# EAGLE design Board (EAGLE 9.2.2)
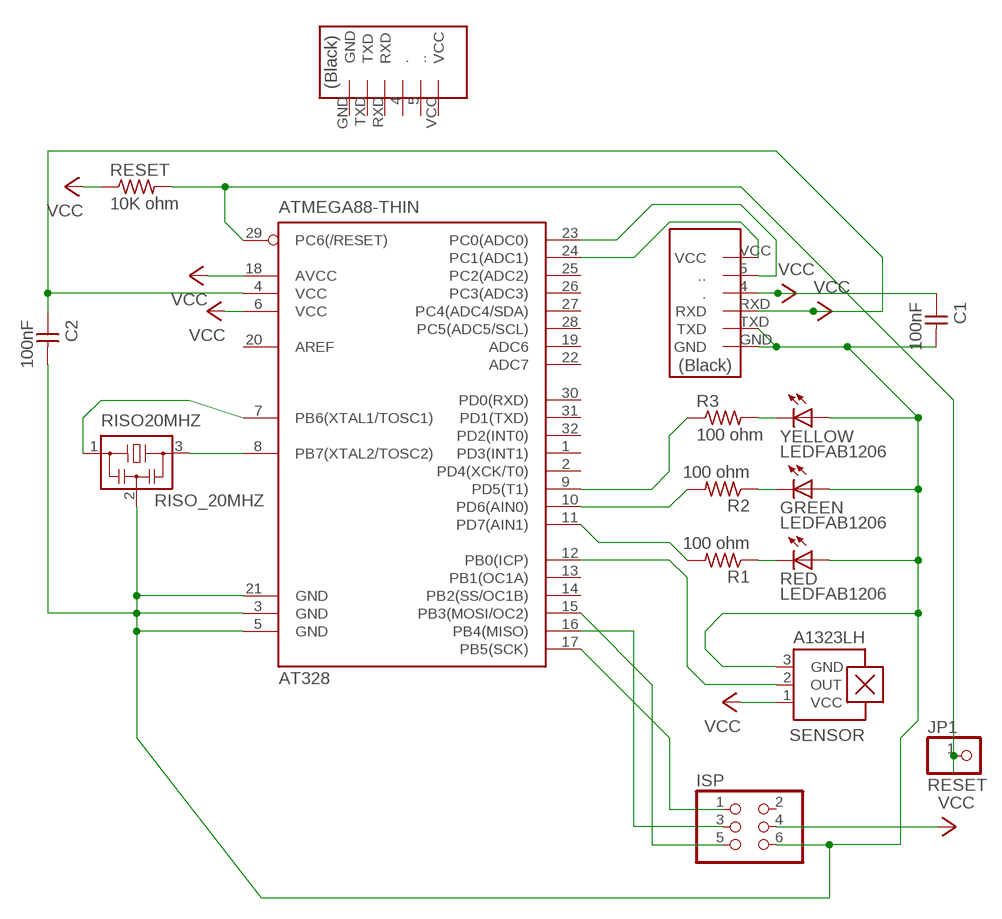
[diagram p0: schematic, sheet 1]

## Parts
AT328  ATMEGA88-THIN  [TQFP32-08THIN]
C1  100nF  CAP-UNPOLARIZEDFAB  [C1206FAB]
C2  100nF  CAP-UNPOLARIZEDFAB  [C1206FAB]
FTDI  FTDI-SMD-HEADER  [1X06SMD]
GREEN  LEDFAB1206  [LED1206FAB]
ISP  PINHD-2X3-SMD  [2X03SMD]
JP1  RESET  PINHD-1X1  [1X01]
R1  100 ohm  RES-US1206FAB  [R1206FAB]
R2  100 ohm  RES-US1206FAB  [R1206FAB]
R3  100 ohm  RES-US1206FAB  [R1206FAB]
RED  LEDFAB1206  [LED1206FAB]
RESET  10K ohm  RES-US1206FAB  [R1206FAB]
RISO20MHZ  RISO_20MHZ  RESONATOR  [EFOBM]
SENSOR  A1323LH  [SOT23-W]
U$1  PINO_FTDI-SMD  [1X06SMD]
YELLOW  LEDFAB1206  [LED1206FAB]

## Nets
GND: AT328.3(GND) AT328.5(GND) AT328.21(GND) C1.2 C2.2 FTDI.GND FTDI.TXD GREEN.1(A) ISP.6(6_GND) RED.1(A) RISO20MHZ.2 SENSOR.3(GND) YELLOW.1(A)
MISO: AT328.16(PB4(MISO)) ISP.3(3_MISO)
MOSI: AT328.15(PB3(MOSI/OC2)) ISP.5(5_MOSI)
N$1: R3.2 YELLOW.2(C)
N$2: R1.1 RED.2(C)
N$3: GREEN.2(C) R2.1
N$4: AT328.11(PD7(AIN1)) R1.2
N$5: AT328.10(PD6(AIN0)) R2.2
N$6: AT328.9(PD5(T1)) R3.1
OUT1: AT328.24(PC1(ADC1)) FTDI.VCC
OUT2: AT328.23(PC0(ADC0)) FTDI.5(..)
OUT_SENSOR: AT328.12(PB0(ICP)) SENSOR.2(OUT)
RESET: AT328.29(PC6(/RESET)) JP1.1 RESET.2
SCK: AT328.17(PB5(SCK)) ISP.1(1_SCK)
VCC: AT328.4(VCC) AT328.6(VCC) AT328.18(AVCC) C1.1 C2.1 FTDI.4(.) FTDI.RXD ISP.4(4_VCC) RESET.1 SENSOR.1(VCC)
XSTAL1: AT328.7(PB6(XTAL1/TOSC1)) RISO20MHZ.1
XSTAL2: AT328.8(PB7(XTAL2/TOSC2)) RISO20MHZ.3
Unconnected: AT328.1(PD3(INT1)) AT328.2(PD4(XCK/T0)) AT328.13(PB1(OC1A)) AT328.14(PB2(SS/OC1B)) AT328.19(ADC6) AT328.20(AREF) AT328.22(ADC7) AT328.25(PC2(ADC2)) AT328.26(PC3(ADC3)) AT328.27(PC4(ADC4/SDA)) AT328.28(PC5(ADC5/SCL)) AT328.30(PD0(RXD)) AT328.31(PD1(TXD)) AT328.32(PD2(INT0)) ISP.2(2_RESET) U$1.4(.) U$1.5(..) U$1.GND U$1.RXD U$1.TXD U$1.VCC

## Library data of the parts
AT328 = fab:ATMEGA88-THIN
C1 C2 = fab:CAP-UNPOLARIZED
FTDI = fab:FTDI-SMD-HEADER
GREEN RED YELLOW = fab:LED: LED
ISP = fab:PINHD-2X3-SMD: PIN HEADER
JP1 = pinhead:PINHD-1X1: PIN HEADER
R1-R3 RESET = fab:RES-US: Resistor (US Symbol)
RISO20MHZ = fab:RESONATOR
SENSOR = allegro:A13*?: Linear Hall Effect Sensor ICs Continuous-Time Ratiometric High-Temperature Operation Programmable Linear with Analog Output A1302 -Replacement- UGN3503 Source: http://www.allegromicro.com/en/Products/Part_Numbers/1301/1301.pdf http://www.allegromicro.com/en/Products/Part_Numbers/1321/1321.pdf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; MF: ALLEGRO MICROSYSTEMS, INC.; MPN: A1323LLHLT-T; OC_FARNELL: 1651968; OC_NEWARK: 65K5152
U$1 = fab:PINO_FTDI-SMD

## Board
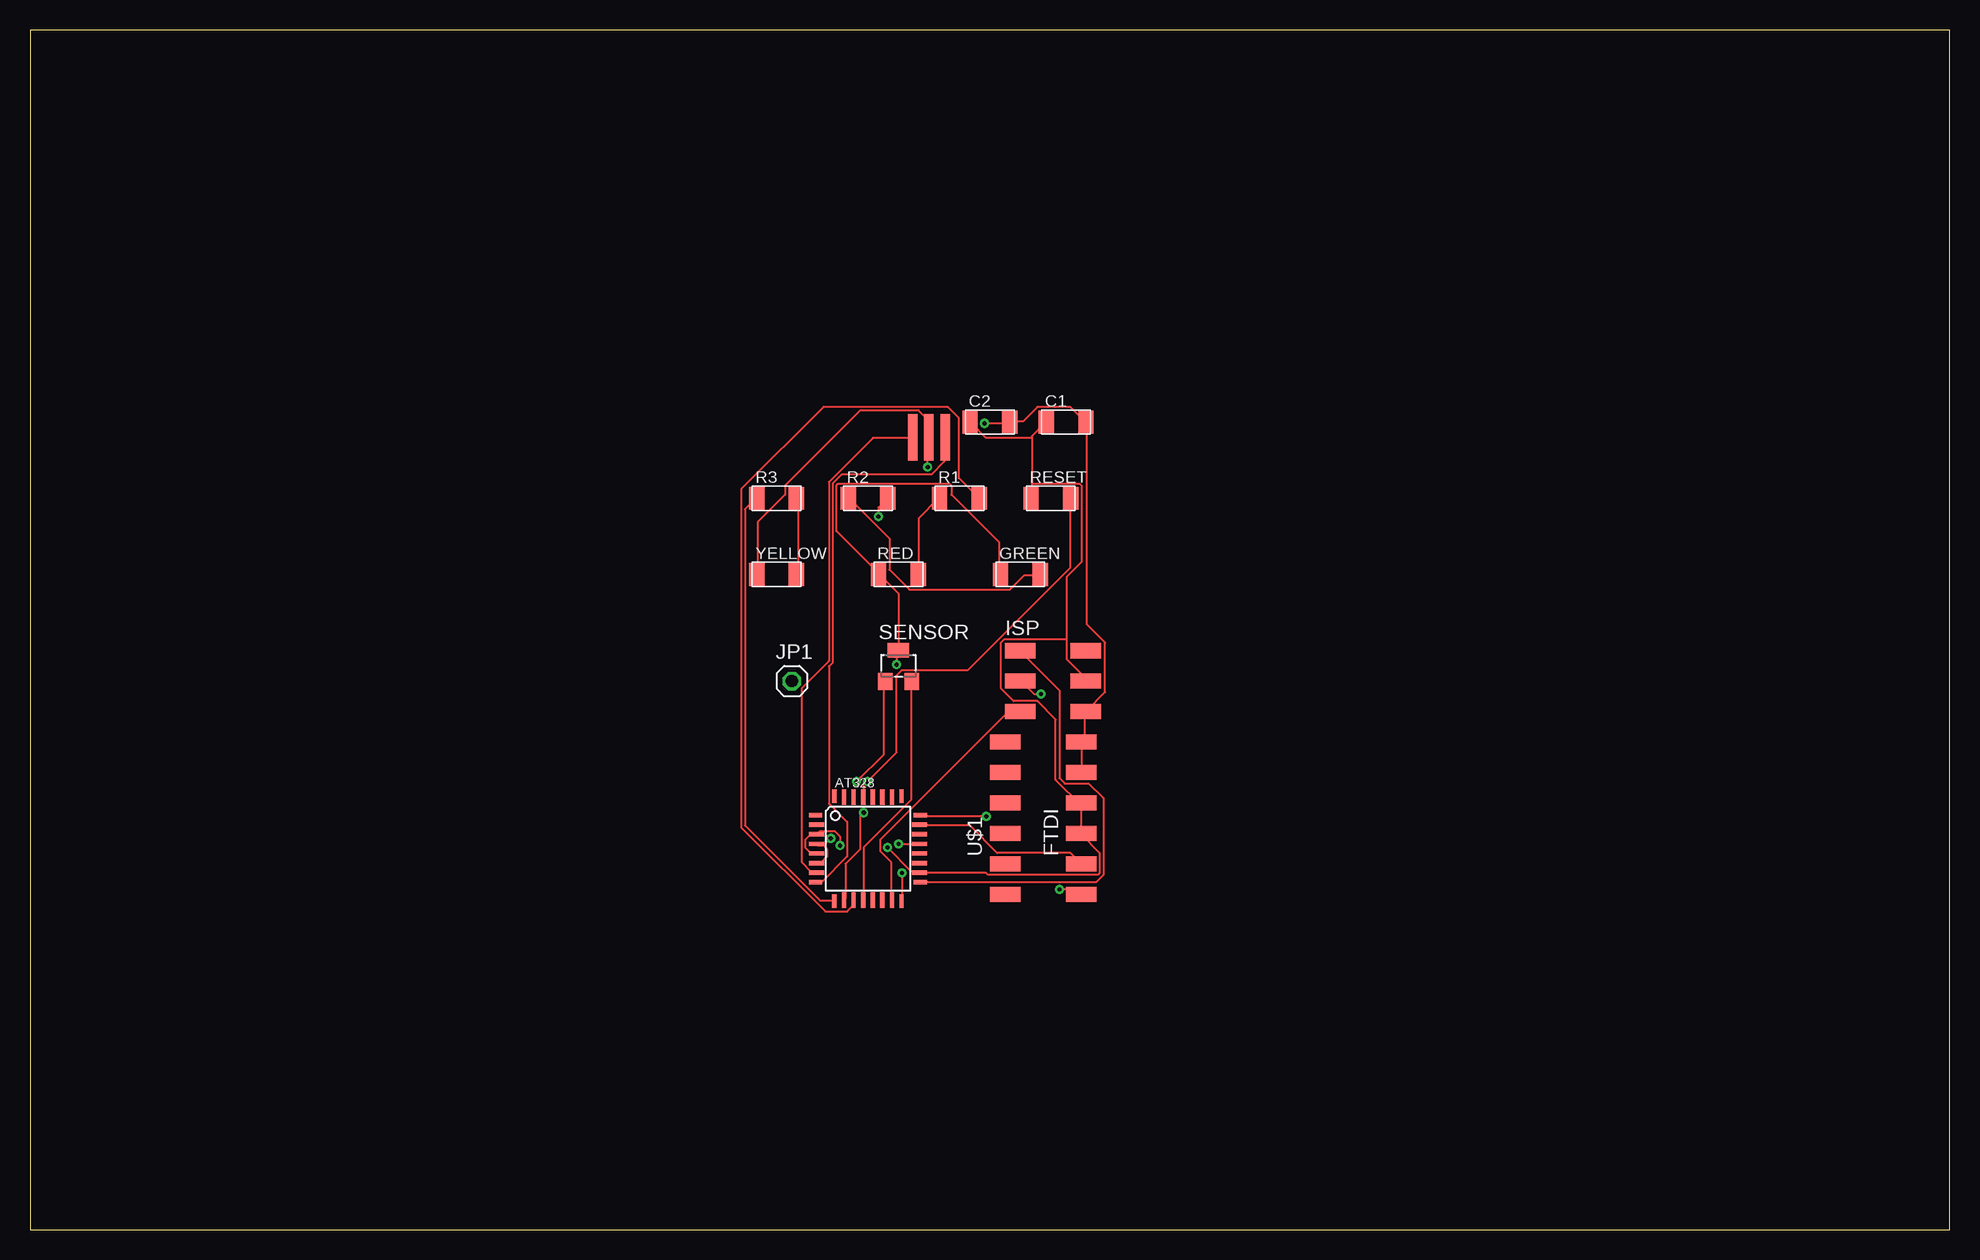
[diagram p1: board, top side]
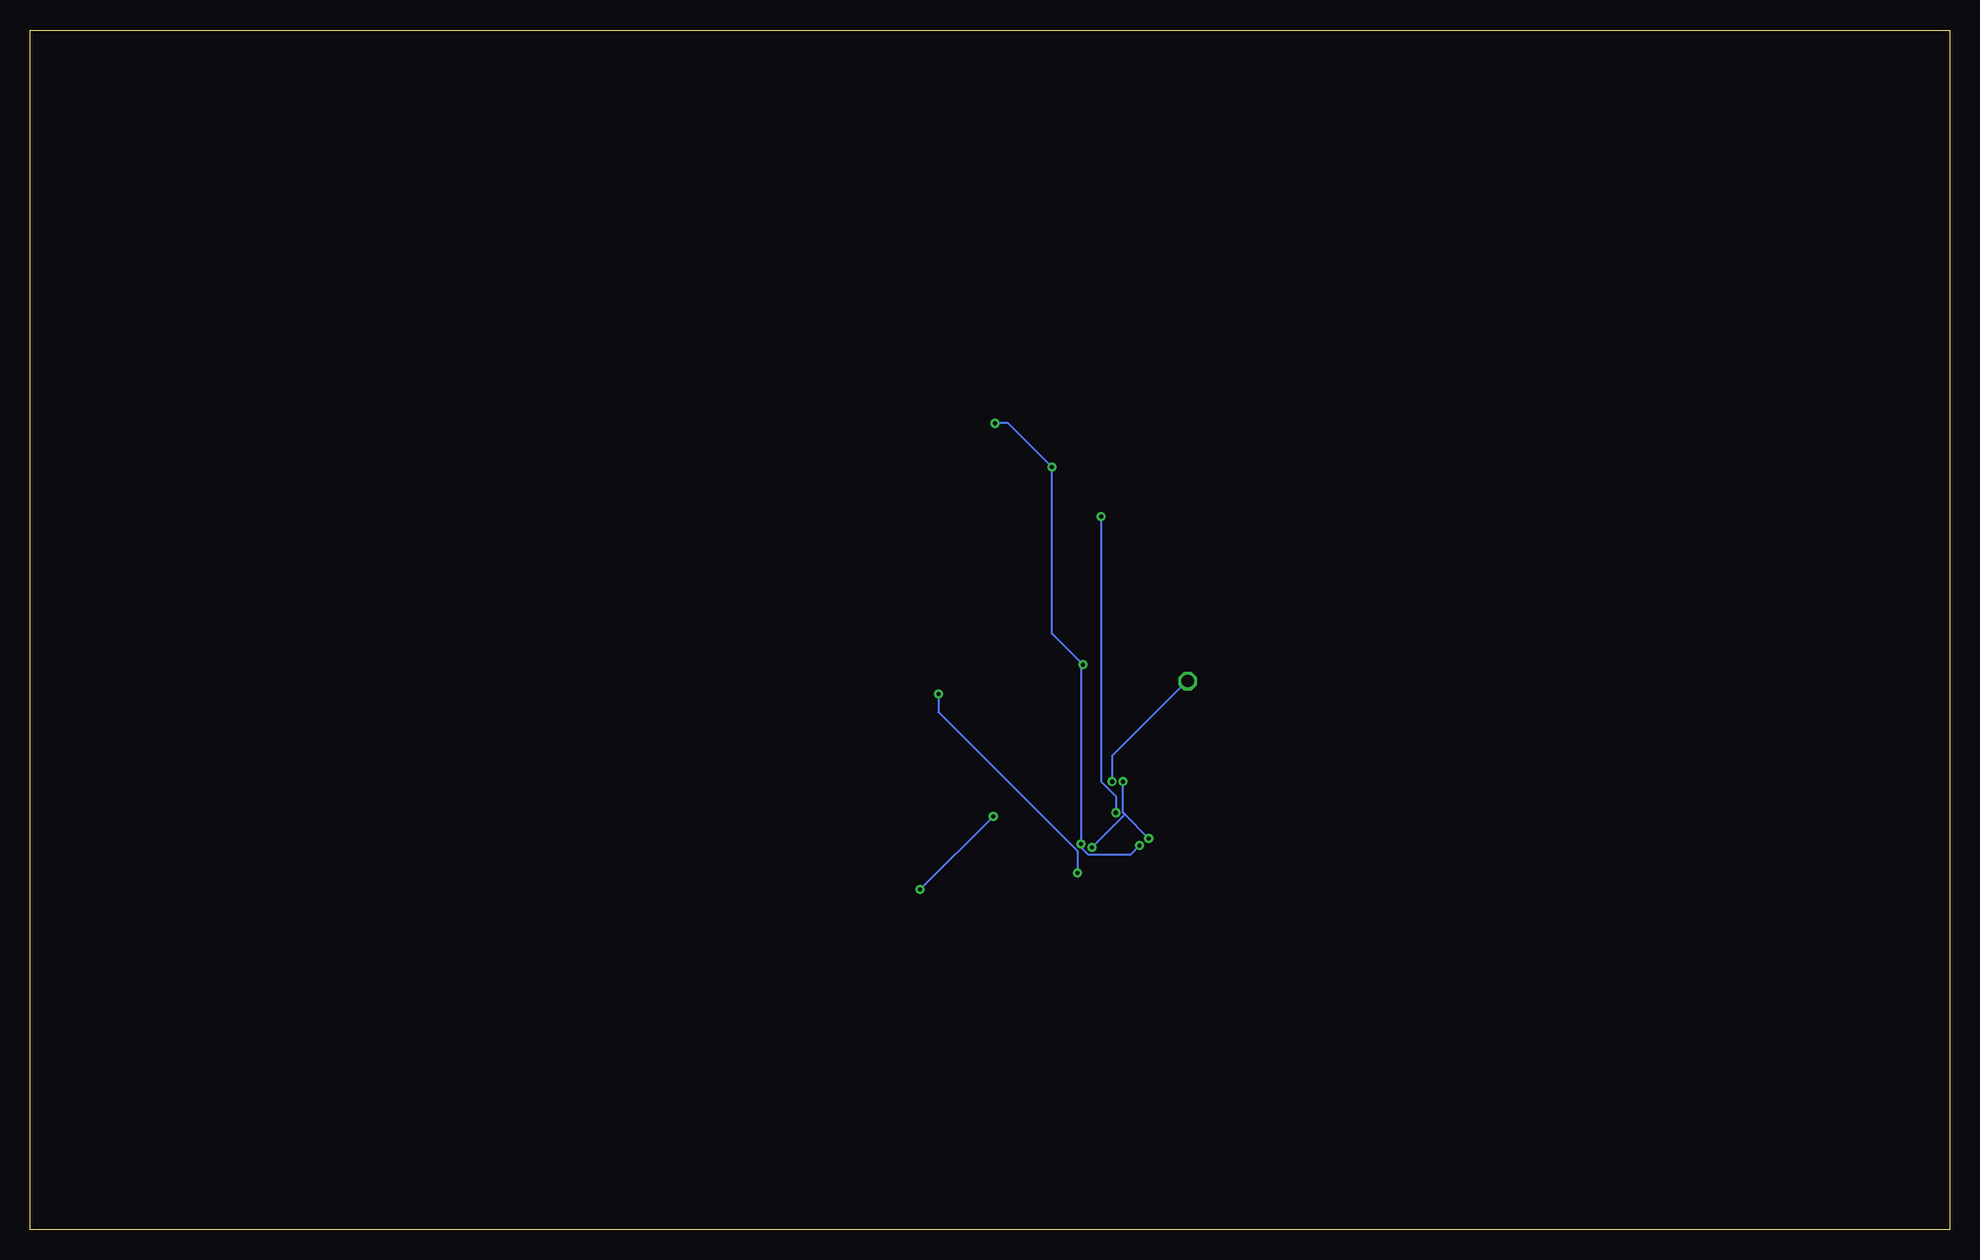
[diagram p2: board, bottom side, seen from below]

Size 160 x 100 mm. Coordinates in mm from the lower left corner, seen from the top.
Outline: 0,0 160,0 160,100 0,100 0,0
Copper layers (1*16): Top 0.035mm / dielectric 1.5mm / Bottom 0.035mm
Design rules "default": minimum track width 6mil, minimum drill 0.35mm, track to track 6mil, track to pad 6mil, pad to pad 6mil, via to via 6mil, smd to smd 6mil, copper to edge 40mil, drill to drill 6mil, minimum pad ring 10mil, minimum via ring 8mil, stop-mask expansion 4mil, vias tented up to drill 0mil, thermal gap 10mil

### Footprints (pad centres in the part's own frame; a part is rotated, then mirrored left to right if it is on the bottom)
TQFP32-08THIN = smd 1.118 x 0.356: 1 -4.369,2.8; 8 -4.369,-2.8; 17 4.369,-2.8; 24 4.369,2.8 | smd 1.27 x 0.356: 2 -4.293,2; 3 -4.293,1.2; 4 -4.293,0.4; 5 -4.293,-0.4; 6 -4.293,-1.2; 7 -4.293,-2; 18 4.293,-2; 19 4.293,-1.2; 20 4.293,-0.4; 21 4.293,0.4; 22 4.293,1.2; 23 4.293,2 | smd 0.356 x 1.118: 9 -2.8,-4.369; 16 2.8,-4.369; 25 2.8,4.369; 32 -2.8,4.369 | smd 0.356 x 1.27: 10 -2,-4.293; 14 1.2,-4.293; 15 2,-4.293; 26 2,4.293; 27 1.2,4.293; 31 -2,4.293 | smd 0.35 x 1.27: 11 -1.2,-4.293; 12 -0.4,-4.293; 13 0.4,-4.293; 28 0.4,4.293; 29 -0.4,4.293; 30 -1.2,4.293
C1206FAB = smd 1.27 x 1.905: 1 -1.651,0; 2 1.651,0
1X06SMD = smd 2.54 x 1.27: 4 0,-1.27; 5 0,-3.81; GND 0,6.35; RXD 0,1.27; TXD 0,3.81; VCC 0,-6.35
LED1206FAB = smd 1.27 x 1.905: 1 -1.651,0; 2 1.651,0
2X03SMD = smd 2.54 x 1.27: 1 -2.54,2.54; 2 2.92,2.54; 3 -2.54,0; 4 2.92,0; 5 -2.54,-2.54; 6 2.92,-2.54
1X01 = drill 1.016 octagon: 1 0,0
R1206FAB = smd 1.27 x 1.905: 1 -1.651,0; 2 1.651,0
EFOBM = smd 0.8 x 3.9: 1 -1.35,0; 2 0,0; 3 1.35,0
SOT23-W = smd 1.2 x 1.4: 1 -1.1,-1.3; 2 1.1,-1.3 | smd 1.8 x 1.2: 3 0,1.3

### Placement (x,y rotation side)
AT328  69.85,31.75 0 top
C1  86.36,67.31 0 top
C2  80.01,67.31 0 top
FTDI  87.63,34.29 0 top
GREEN  82.55,54.61 0 top
ISP  85.09,45.72 0 top
JP1  63.5,45.72 0 top
R1  77.47,60.96 0 top
R2  69.85,60.96 0 top
R3  62.23,60.96 0 top
RED  72.39,54.61 0 top
RESET  85.09,60.96 0 top
RISO20MHZ  74.93,66.04 0 top
SENSOR  72.39,46.99 0 top
U$1  81.28,34.29 0 top
YELLOW  62.23,54.61 0 top

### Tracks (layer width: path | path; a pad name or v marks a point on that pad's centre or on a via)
GND  (via drill 0.35)
  Top 0.152: FTDI.TXD FTDI.GND 87.63,40.69 87.94,41 87.94,43.13 ISP.6 88.09,43.28 89.61,44.81 89.61,48.92 88.09,50.44 88.09,67.21 C1.2 87.94,67.36 86.72,68.58 83.97,68.58 82.75,67.36 81.69,67.36 C2.2 81.53,67.21 v79.55,67.21 | YELLOW.1 60.66,54.71 60.66,58.98 62.94,61.27 62.94,62.03 69.19,68.28 74.07,68.28 74.83,67.51 74.83,66.14 RISO20MHZ.2 74.83,65.99 v74.83,63.55 | AT328.5 65.53,31.39 65.08,31.39 64.62,31.85 64.62,32.46 65.08,32.92 65.53,32.92 AT328.3 65.68,33.07 65.84,33.22 67.06,33.22 67.51,32.77 v67.51,32 | v72.39,32.16 74.07,32.16 AT328.21 | GREEN.1 80.77,54.71 80.77,57.3 76.81,61.27 76.81,62.03 76.66,62.18 67.36,62.18 67.21,62.03 67.21,58.22 70.71,54.71 RED.1 70.87,54.56 72.39,53.03 SENSOR.3 72.39,48.16 72.24,48.01 v72.24,47.09
  Bottom 0.152: v67.51,32 68.28,31.24 71.78,31.24 72.39,31.85 v72.39,32.16 72.39,46.94 v72.24,47.09 74.83,49.68 v74.83,63.55 78.49,67.21 v79.55,67.21
MISO  (via drill 0.35)
  Top 0.152: v72.69,29.72 72.69,27.43 AT328.16 | v84.28,44.65 83.67,44.65 82.6,45.72 ISP.3
  Bottom 0.152: v72.69,29.72 72.69,31.55 84.28,43.13 v84.28,44.65
MOSI
  Top 0.152: AT328.15 71.78,27.58 71.78,30.63 70.87,31.55 70.87,32.46 81.53,43.13 82.45,43.13 ISP.5
N$1
  Top 0.152: YELLOW.2 64.01,54.71 64.01,60.96 R3.2
N$2
  Top 0.152: RED.2 74.07,54.71 74.07,59.28 75.74,60.96 R1.1
N$3
  Top 0.152: GREEN.2 84.12,54.56 82.91,54.56 81.69,53.34 73.3,53.34 71.63,55.02 71.63,57.61 68.28,60.96 R2.1
N$4
  Top 0.152: AT328.11 68.58,27.43 68.58,26.98 68.12,26.52 66.29,26.52 59.28,33.53 59.28,61.72 66.14,68.58 76.5,68.58 77.42,67.67 77.42,62.64 79.1,60.96 R1.2
N$5  (via drill 0.35)
  Top 0.152: v69.49,34.75 69.19,34.44 69.19,31.7 67.97,30.48 67.97,27.58 AT328.10 | v70.71,59.44 70.71,60.2 71.48,60.96 R2.2
  Bottom 0.152: v69.49,34.75 69.49,36.12 70.71,37.34 v70.71,59.44
N$6
  Top 0.152: AT328.9 66.9,27.43 65.84,27.43 59.59,33.68 59.59,60.05 60.5,60.96 R3.1
OUT1  (via drill 0.35)
  Top 0.152: v79.7,34.44 74.22,34.44 AT328.24 | v85.8,28.35 87.33,28.35 87.63,28.04 FTDI.VCC
  Bottom 0.152: v85.8,28.35 v79.7,34.44
OUT2
  Top 0.152: FTDI.5 86.72,31.39 80.62,31.39 78.33,33.68 74.22,33.68 AT328.23
OUT_SENSOR
  Top 0.152: AT328.12 69.49,27.58 69.49,31.85 73.46,35.81 73.46,45.57 SENSOR.2
RESET  (via drill 0.35)
  Top 0.152: AT328.29 69.49,36.12 69.49,37.03 v69.8,37.34 72.24,39.78 72.24,46.18 72.69,46.63 78.18,46.63 86.72,55.17 86.72,60.96 RESET.2
  Bottom 0.152: v69.8,37.34 69.8,39.47 63.55,45.72 JP1.1
SCK
  Top 0.152: AT328.17 88.85,28.96 89.46,29.57 89.46,35.97 88.24,37.19 86.26,37.19 85.8,37.64 85.8,44.96 82.6,48.16 ISP.1
VCC  (via drill 0.35)
  Top 0.152: 83.52,65.99 83.52,66.14 84.58,67.21 C1.1 | 83.52,65.99 83.52,62.18 | 83.52,62.18 83.52,60.96 RESET.1 | 83.52,65.99 79.7,65.99 78.49,67.21 C2.1 | 86.41,49.23 86.41,54.41 87.63,55.63 87.63,62.03 87.48,62.18 83.52,62.18 | 86.41,49.23 86.41,47.55 87.94,46.02 87.94,45.72 ISP.4 | 66.14,32 66.45,31.7 66.45,31.09 65.99,30.63 65.68,30.63 AT328.6 | 66.14,32 65.68,32 AT328.4 66.14,32 | v68.89,37.34 71.17,39.62 71.17,45.57 SENSOR.1 | 66.14,32 v66.75,32.61 | 87.63,35.36 FTDI.4 87.63,32.92 89.15,31.39 89.15,29.72 89,29.57 79.86,29.57 79.7,29.72 74.22,29.72 AT328.18 74.07,29.87 73.46,29.87 v71.48,31.85 | 87.63,35.36 FTDI.RXD 87.63,35.51 | 86.41,49.23 81.23,49.23 80.92,48.92 80.92,45.11 81.99,44.04 83.97,44.04 85.5,42.52 85.5,37.49 87.63,35.36
  Bottom 0.152: v68.89,37.34 68.89,34.75 68.73,34.59 | v66.75,32.61 68.73,34.59 | v71.48,31.85 68.73,34.59
XSTAL1
  Top 0.152: AT328.7 65.53,29.87 65.08,29.87 64.31,30.63 64.31,45.11 66.6,47.4 66.6,62.33 70.26,65.99 73.46,65.99 RISO20MHZ.1
XSTAL2
  Top 0.152: AT328.8 65.53,28.96 65.99,28.96 68.12,31.09 68.12,33.98 66.6,35.51 66.6,46.94 66.9,47.24 66.9,62.18 67.67,62.94 75.13,62.94 76.2,64.01 76.2,65.99 RISO20MHZ.3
